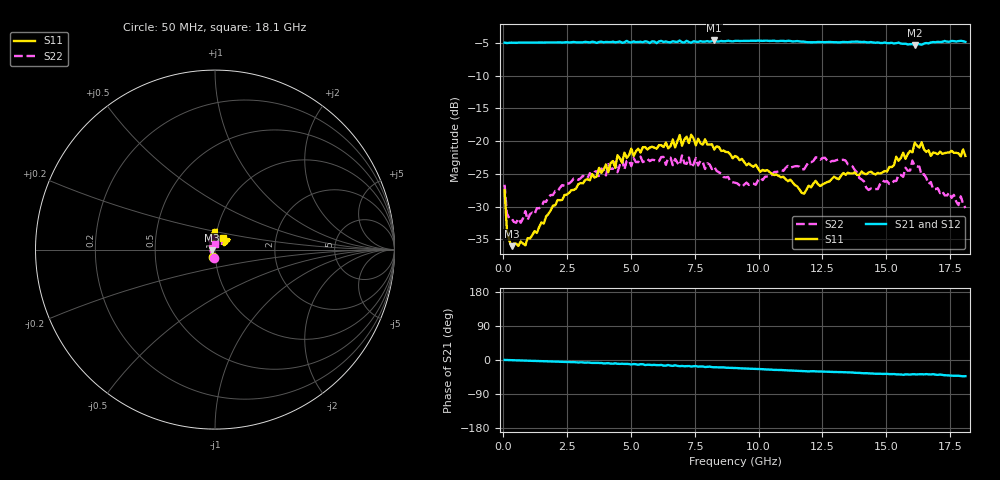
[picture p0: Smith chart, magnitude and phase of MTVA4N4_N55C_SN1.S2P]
! Network Analyzer HP8720D.06.14 Serial No. US36140669
! 28 Jun 2005  10:10:22
! Frequency  S11  S21  S12  S22
# HZ  S  DB R 50
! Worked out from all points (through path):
!   201 points, 50 MHz to 18.1 GHz, reference 50 ohm
!   highest |S21| = -4.65 dB at 8.263 GHz (marker M1); lowest = -5.3 dB at 16.11 GHz (marker M2)
!   group delay of S21, straight-line fit = 6.8 ps
!   lowest |S11| = -36.0 dB at 320.8 MHz (marker M3), VSWR 1.03, Z = 48.5 - j0.418 ohm
!   |S11| at or under -10 dB: start of sweep to end of sweep
!   |S22| runs from -32.5 to -22.2 dB; largest |S21 - S12| = 0.017
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5e7  -27.51 -104.0  -4.98 0.1  -5.00 0.3  -26.67 -95.1
1.4025e8  -33.58 -130.6  -5.04 -0.1  -5.03 -0.0  -31.09 -143.4
3.2075e8  -36.04 -164.1  -4.98 -0.3  -5.00 -0.4  -31.78 -168.5
8.6225e8  -35.92 146.7  -4.98 -1.6  -4.99 -1.5  -30.68 164.6
9.525e8  -34.82 144.6  -4.97 -1.6  -4.98 -1.7  -32.04 157.9
2.12575e9  -29.00 102.2  -4.94 -4.5  -4.95 -4.4  -27.69 122.3
3.1185e9  -26.46 97.5  -4.93 -6.4  -4.94 -6.7  -25.29 123.3
4.382e9  -24.08 88.1  -4.93 -8.8  -4.88 -9.8  -23.19 115.7
4.47225e9  -22.16 84.0  -4.90 -9.9  -4.86 -9.2  -24.76 118.2
4.65275e9  -23.31 84.0  -4.99 -9.8  -4.83 -10.3  -22.79 116.5
6.09675e9  -20.62 88.0  -4.78 -13.5  -4.73 -13.5  -23.06 101.8
6.99925e9  -20.72 90.1  -4.92 -15.7  -4.95 -16.8  -22.17 93.7
7.36025e9  -19.03 84.2  -4.99 -17.1  -4.86 -16.5  -24.00 97.5
8.26275e9  -21.30 97.0  -4.65 -19.2  -4.75 -19.6  -23.91 83.6
9.075e9  -22.27 101.9  -4.71 -21.1  -4.70 -21.2  -26.35 75.0
1.169225e10  -27.92 86.3  -4.82 -29.5  -4.81 -29.5  -24.32 62.6
1.21435e10  -26.49 81.0  -4.92 -29.5  -4.88 -29.8  -23.05 69.1
1.3407e10  -25.14 53.7  -4.89 -32.4  -4.86 -32.6  -22.99 70.6
1.43095e10  -24.81 30.9  -4.94 -35.3  -4.91 -35.7  -27.47 76.7
1.512175e10  -23.95 28.6  -5.05 -37.3  -4.96 -37.2  -26.55 72.2
1.61145e10  -20.23 35.7  -5.33 -37.6  -5.11 -38.2  -23.82 52.1
1.81e10  -22.26 55.0  -4.86 -42.7  -4.91 -43.7  -30.22 91.1
